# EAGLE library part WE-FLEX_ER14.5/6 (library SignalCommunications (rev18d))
WE-FLEX Flexible Transformer for DC/DC Converter Characteristics Transformer with 6 identical windings 4 sizes with 5 different lengths of air gap each Insulation test voltage 500 VAC Low leakage inductance Operating temperature: –40 ºC to +125 ºC By using different circuits more than 375 transformer solutions and about 125 choke solutions possible. Consequently, quick prototyping possibilities Applications All kind of switching regulators -Flyback converters -Forward converters -Push-pull converters -Step-up/step-down converters -SEPIC converter Details see: http://katalog.we-online.de/en/pbs/WE-FLEX? Updated by Dan Xu 2014-07-07 2014 (C) Wurth Elektronik
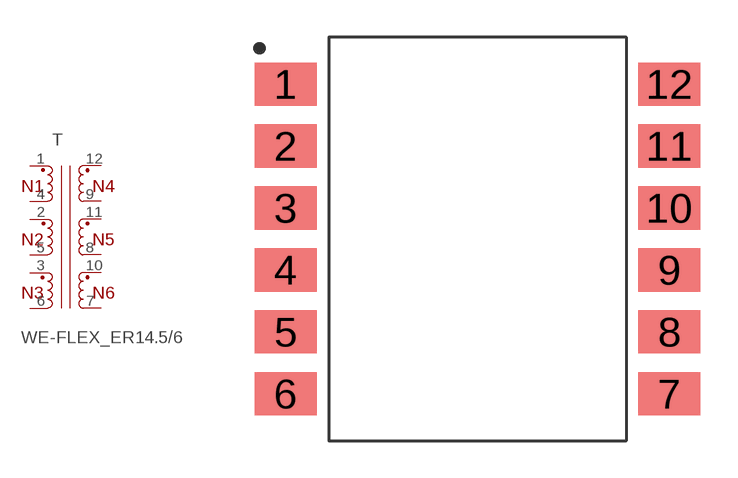
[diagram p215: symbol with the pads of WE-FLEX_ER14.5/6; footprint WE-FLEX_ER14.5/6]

Designator prefix T

## WE-FLEX_ER14.5/6_749196201, WE-FLEX_ER14.5/6_749196211, WE-FLEX_ER14.5/6_749196221, WE-FLEX_ER14.5/6_749196231, WE-FLEX_ER14.5/6_749196241  [WE-FLEX_ER14.5/6]
1  1  pas
2  11  pas
3  9  pas
4  12  pas
5  10  pas
6  8  pas
7  7  pas
8  5  pas
9  3  pas
10  6  pas
11  4  pas
12  2  pas

## Footprint WE-FLEX_ER14.5/6 (pad centres in mm)
smd 2.5 x 1.75: 1 -7.75,6.25; 2 -7.75,3.75; 3 -7.75,1.25; 4 -7.75,-1.25; 5 -7.75,-3.75; 6 -7.75,-6.25; 7 7.75,-6.25; 8 7.75,-3.75; 9 7.75,-1.25; 10 7.75,1.25; 11 7.75,3.75; 12 7.75,6.25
